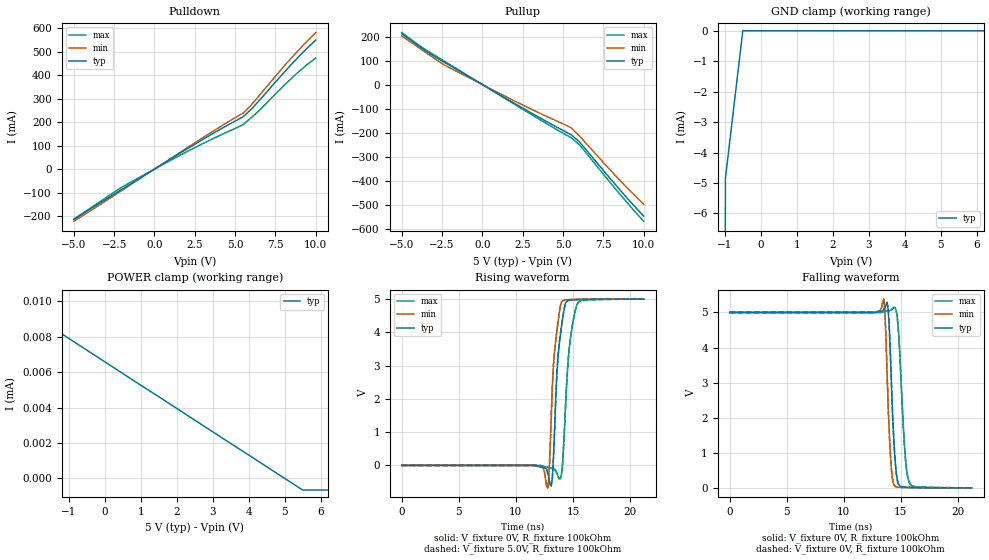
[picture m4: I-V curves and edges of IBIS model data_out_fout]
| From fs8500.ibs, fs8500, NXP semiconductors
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|   Model data_out_fout
[Model]   data_out_fout
Model_type   Output
Polarity   Non-Inverting
Vmeas = 2.5
Cref = 0pF
Rref = 50
|   typ   min   max
C_comp   2.949p  2.447p  4.788p
|   typ min max
[Power Clamp Reference]  5.0 NA NA
[GND Clamp Reference]   0   NA NA
[pullup reference]   5.0 NA NA
[pulldown reference]   0   NA NA
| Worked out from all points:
|   slope of the pulldown table from 0 to 0.75 V, typ, clamps not added: 23.4 ohm
|   slope of the pullup table from 0 to 0.75 V, typ, clamps not added: 25.4 ohm
|   rising waveform, V_fixture 0V, R_fixture 100kOhm: 20-80 % time 542ps typ, 523ps min, 611ps max; typ from 0 V to 5 V
|   falling waveform, V_fixture 0V, R_fixture 100kOhm: 20-80 % time 396ps typ, 355ps min, 488ps max; typ from 5 V to 0 V
|   rising waveform, V_fixture 5.0V, R_fixture 100kOhm: 20-80 % time 541ps typ, 522ps min, 611ps max; typ from 0.001 V to 5 V
|   falling waveform, V_fixture 0V, R_fixture 100kOhm: 20-80 % time 396ps typ, 356ps min, 488ps max; typ from 5 V to 0.001 V
[GND Clamp]
|Voltage   I(typ)   I(min)   I(max)
-5V       -4.5A      NA         NA
-1.267V   -210mA     NA         NA
-984mV    -4.86mA    NA         NA
-500mV    -562pA     NA         NA
10V       909pA      NA         NA
[POWER Clamp]
|Voltage   I(typ)   I(min)   I(max)
-5V       3A         NA         NA
-2.42V    505uA      NA         NA
-1.944V   9.14uA     NA         NA
5.5V      -658nA     NA         NA
10V       -658nA     NA         NA
|   typ   min   max
[Temperature Range]   27   -40   175
[Pulldown]
|Voltage   I(typ)   I(min)   I(max)
-5V       -215.6mA   -222.2mA   -212.3mA
-2.5V     -107mA     -112.4mA   -98.17mA
-1.5V     -64.38mA   -67.47mA   -56.74mA
2.5V      105.7mA    111.6mA    91.32mA
5.5V      222.8mA    238.8mA    189.5mA
6V        254.8mA    273.1mA    218.4mA
6.5V      291.9mA    313.1mA    249.8mA
8.5V      446.2mA    474mA      386.7mA
9.5V      516.7mA    547.1mA    446.9mA
10V       549.2mA    581.1mA    472.6mA
[Pullup]
|Voltage   I(typ)   I(min)   (max)
-5V       211.3mA    201.9mA    216.4mA
-3.5V     138.9mA    132.9mA    144mA
-2.5V     98.27mA    87.25mA    103mA
-2V       78.76mA    68.74mA    82.5mA
2.5V      -97.85mA   -84.92mA   -102.8mA
5.5V      -208.5mA   -179.5mA   -221.1mA
6V        -237.1mA   -212.5mA   -249.3mA
8.5V      -436mA     -396.4mA   -454mA
10V       -547.1mA   -497.5mA   -568.8mA
[Ramp]
R_load = 100kohm
|   typ   min   max
dV/dt_r   4.955/1e-9   4.277/1e-9   5.236/1e-9
dV/dt_f   6.882/1e-9   5.485/1e-9   7.724/1e-9
[Rising Waveform]
V_fixture = 0V
R_fixture = 100kOhm
|Time   V(typ)   V(min)   V(max)
0s        2.61nV     264pV      1.48uV
12.8ns    -240mV     -675mV     -58.3mV
13.1ns    -617mV     1.466V     -78.4mV
13.4ns    1.14V      3.47V      -119mV
13.6ns    2.807V     4.069V     -241mV
14ns      4.19V      4.913V     -262mV
14.4ns    4.909V     4.978V     2.135V
14.8ns    4.973V     4.987V     3.87V
15.5ns    4.987V     4.993V     4.914V
21.2ns    4.999V     4.999V     4.998V
[falling Waveform]
V_fixture = 0V
R_fixture = 100kOhm
|Time   V(typ)   V(min)   V(max)
0s        4.999V     4.999V     4.999V
13.5ns    5.078V     5.378V     5.018V
13.6ns    5.132V     5.012V     5.027V
13.9ns    5.033V     2.18V      5.04V
14.2ns    2.694V     417mV      5.085V
14.4ns    1.25V      79.3mV     5.145V
14.7ns    195mV      21mV       4.802V
15.3ns    20.4mV     10.1mV     1.262V
15.7ns    14mV       7.06mV     185mV
21.2ns    78.2uV     13.9uV     1.21mV
[Rising Waveform]
V_fixture = 5.0V
R_fixture = 100kOhm
|Time   V(typ)   V(min)   V(max)
0s        1.16mV     1.11mV     1.32mV
12.8ns    -237mV     -672mV     -56.9mV
13.1ns    -614mV     1.47V      -76.8mV
13.4ns    1.14V      3.473V     -116mV
13.6ns    2.814V     4.072V     -237mV
14ns      4.192V     4.915V     -259mV
14.4ns    4.911V     4.979V     2.14V
14.8ns    4.975V     4.989V     3.873V
15.5ns    4.989V     4.994V     4.917V
21.2ns    5V         5V         4.999V
[falling Waveform]
V_fixture = 0V
R_fixture = 100kOhm
|Time   V(typ)   V(min)   V(max)
0s        5V         5V         5V
13.5ns    5.08V      5.379V     5.02V
13.6ns    5.133V     5.013V     5.028V
13.9ns    5.033V     2.18V      5.042V
14.2ns    2.692V     418mV      5.087V
14.4ns    1.25V      80.5mV     5.147V
14.7ns    196mV      22.2mV     4.804V
15.3ns    22mV       11.2mV     1.264V
15.7ns    15.4mV     8.15mV     187mV
21.2ns    1.23mV     1.13mV     2.53mV
